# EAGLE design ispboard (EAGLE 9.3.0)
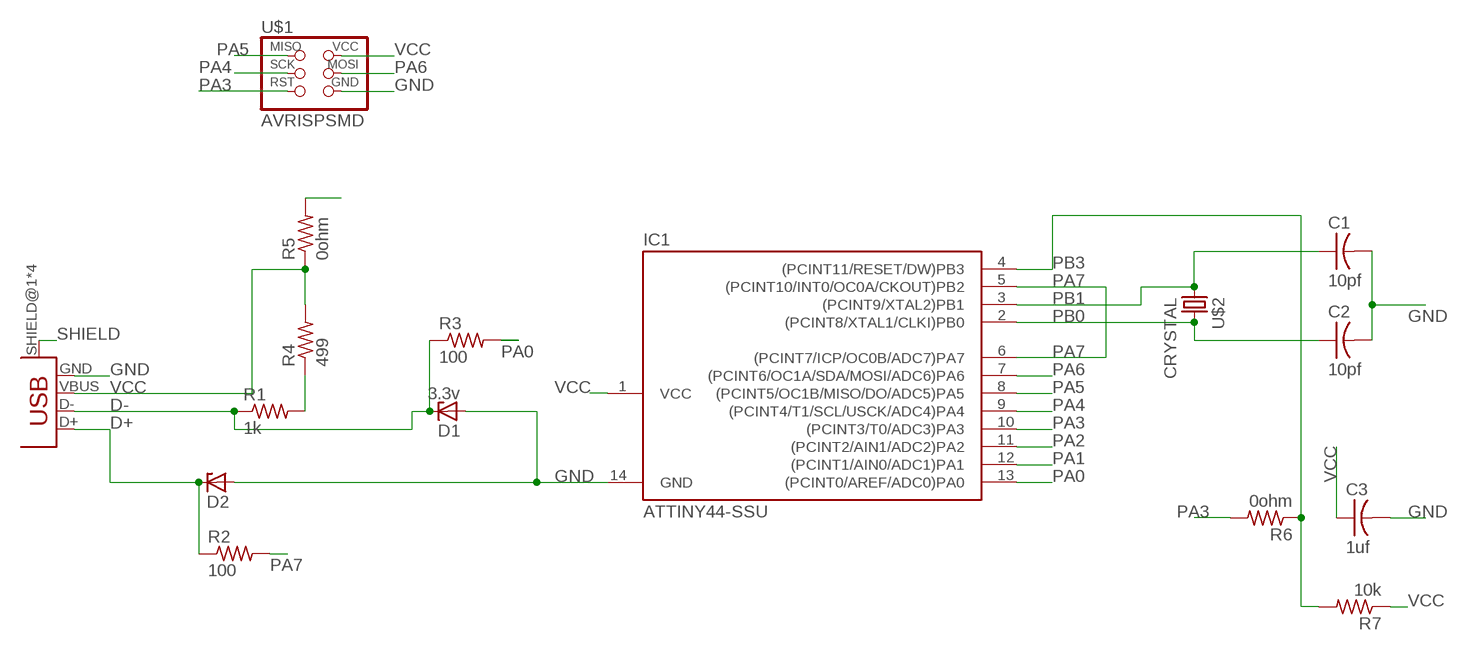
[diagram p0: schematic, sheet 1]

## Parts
C1  10pf  CAP-US1206FAB  [C1206FAB]
C2  10pf  CAP-US1206FAB  [C1206FAB]
C3  1uf  CAP-US1206FAB  [C1206FAB]
D1  3.3v  ZENER_DIODESOD123  [SOD123]
D2  ZENER_DIODESOD123  [SOD123]
IC1  ATTINY44-SSU  [SOIC14]
R1  1k  RES-US1206FAB  [R1206FAB]
R2  100  RES-US1206FAB  [R1206FAB]
R3  100  RES-US1206FAB  [R1206FAB]
R4  499  RES-US1206FAB  [R1206FAB]
R5  0ohm  RES-US1206FAB  [R1206FAB]
R6  0ohm  RES-US1206FAB  [R1206FAB]
R7  10k  RES-US1206FAB  [R1206FAB]
U$1  AVRISPSMD  [2X03SMD]
U$2  CRYSTAL  [2-SMD-5X3MM]
U$3  USB_MINIB  [USB_MINIB]

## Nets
D+: D2.CATHODE R2.1 U$3.D+
D-: D1.CATHODE R1.1 R3.1 U$3.D-
GND: C1.2 C2.2 C3.2 D1.ANODE D2.ANODE IC1.14(GND) U$1.6(GND) U$3.GND
N$1: R1.2 R4.1
PA0: IC1.13((PCINT0/AREF/ADC0)PA0) R3.2
PA1: IC1.12((PCINT1/AIN0/ADC1)PA1)
PA2: IC1.11((PCINT2/AIN1/ADC2)PA2)
PA3: IC1.10((PCINT3/T0/ADC3)PA3) R6.2 U$1.5(RST)
PA4: IC1.9((PCINT4/T1/SCL/USCK/ADC4)PA4) U$1.3(SCK)
PA5: IC1.8((PCINT5/OC1B/MISO/DO/ADC5)PA5) U$1.1(MISO)
PA6: IC1.7((PCINT6/OC1A/SDA/MOSI/ADC6)PA6) U$1.4(MOSI)
PA7: IC1.5((PCINT10/INT0/OC0A/CKOUT)PB2) IC1.6((PCINT7/ICP/OC0B/ADC7)PA7) R2.2
PB0: C2.1 IC1.2((PCINT8/XTAL1/CLKI)PB0) U$2.P$2
PB1: C1.1 IC1.3((PCINT9/XTAL2)PB1) U$2.P$1
PB3: IC1.4((PCINT11/RESET/DW)PB3) R6.1 R7.2
SHIELD: U$3.SHIELD@1(SHIELD) U$3.SHIELD@2(SHIELD) U$3.SHIELD@3(SHIELD) U$3.SHIELD@4(SHIELD)
VCC: C3.1 IC1.1(VCC) R4.2 R5.1 R5.2 R7.1 U$1.2(VCC) U$3.VBUS

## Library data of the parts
C1-C3 = fab:CAP-US
D1 D2 = fab:ZENER_DIODE: zener diode
IC1 = fab:ATTINY44
R1-R7 = fab:RES-US: Resistor (US Symbol)
U$1 = fab:AVRISP
U$2 = fab:CRYSTAL
U$3 = fab:USB_MINIB

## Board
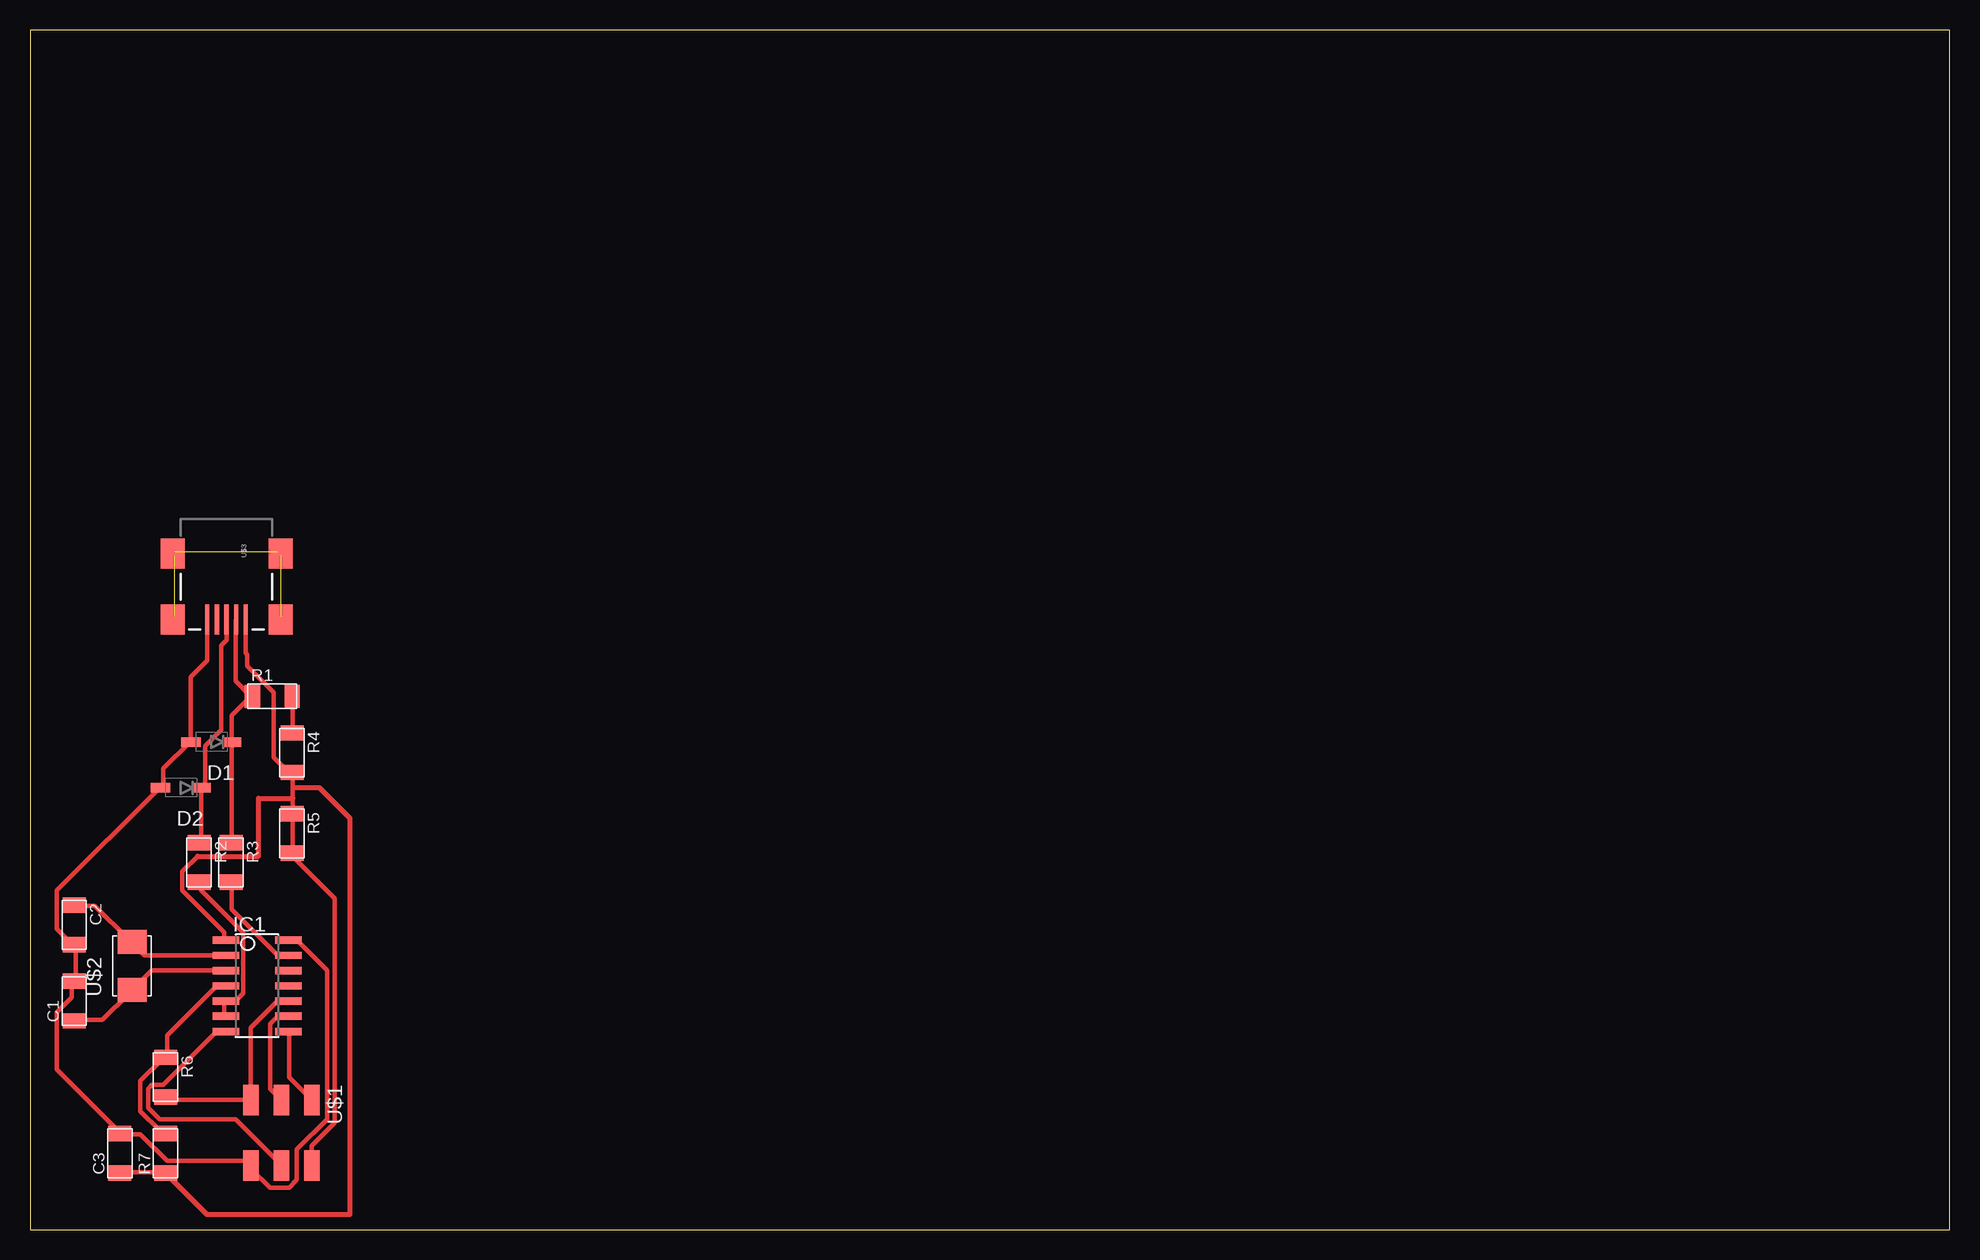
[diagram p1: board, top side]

Size 160 x 100 mm. Coordinates in mm from the lower left corner, seen from the top.
Outline: 0,0 160,0 160,100 0,100 0,0
Copper layers (1*16): Top 0.035mm / dielectric 1.5mm / Bottom 0.035mm
Design rules "default *": minimum track width 15mil, minimum drill 0.35mm, track to track 10mil, track to pad 6mil, pad to pad 6mil, via to via 6mil, smd to smd 6mil, copper to edge 40mil, drill to drill 6mil, minimum pad ring 10mil, minimum via ring 8mil, stop-mask expansion 4mil, vias tented up to drill 0mil, thermal gap 10mil

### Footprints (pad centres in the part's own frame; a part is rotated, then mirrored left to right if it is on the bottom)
C1206FAB = smd 1.27 x 1.905: 1 -1.651,0; 2 1.651,0
SOD123 = smd 1.6 x 0.8: ANODE 1.7,0; CATHODE -1.7,0
SOIC14 = smd 0.61 x 2.21: 1 -3.81,-2.603; 2 -2.54,-2.603; 3 -1.27,-2.603; 4 0,-2.603; 5 1.27,-2.603; 6 2.54,-2.603; 7 3.81,-2.603; 8 3.81,2.603; 9 2.54,2.603; 10 1.27,2.603; 11 0,2.603; 12 -1.27,2.603; 13 -2.54,2.603; 14 -3.81,2.603
R1206FAB = smd 1.27 x 1.905: 1 -1.651,0; 2 1.651,0
2X03SMD = smd 2.54 x 1.27: 1 -2.54,2.54; 2 2.92,2.54; 3 -2.54,0; 4 2.92,0; 5 -2.54,-2.54; 6 2.92,-2.54
2-SMD-5X3MM = smd 2 x 2.4: P$1 -2,0; P$2 2,0
USB_MINIB = smd 2.5 x 0.35: D+ 3.77,0; D- 3.77,0.8; GND 3.77,-1.6; ID 3.77,-0.8; VBUS 3.77,1.6 | smd 2.5 x 2: SHIELD@1 -1.73,-4.5; SHIELD@2 -1.73,4.5; SHIELD@3 3.77,4.5; SHIELD@4 3.77,-4.5

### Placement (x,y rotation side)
C1  3.68,19.05 90 top
C2  3.68,25.4 270 top
C3  7.49,6.35 90 top
D1  15.11,40.64 180 top
D2  12.57,36.83 180 top
IC1  18.92,20.32 270 top
R1  20.19,44.45 0 top
R2  14.1,30.61 270 top
R3  16.76,30.61 270 top
R4  21.84,39.75 270 top
R5  21.84,33.02 270 top
R6  11.3,12.7 270 top
R7  11.3,6.35 90 top
U$1  20.95,8.26 270 top
U$2  8.51,21.97 90 top
U$3  16.38,54.61 270 top

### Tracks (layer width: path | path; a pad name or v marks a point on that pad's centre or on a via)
D+
  Top 0.381: 14.29,36.83 14.29,32.38 R2.1 | 14.29,36.83 14.61,37.15 14.61,40.32 15.94,41.66 15.94,48.7 16.38,49.15 U$3.D+ | 14.29,36.83 D2.CATHODE
D-
  Top 0.381: 16.83,40.64 16.83,42.86 18.41,44.45 | 16.83,40.64 16.83,32.38 R3.1 | 16.83,40.64 D1.CATHODE | 18.41,44.45 17.14,45.72 17.14,50.8 U$3.D- | 18.41,44.45 R1.1
GND
  Top 0.381: D1.ANODE 13.34,40.64 11.11,38.42 11.11,36.83 D2.ANODE 10.79,36.83 2.22,28.26 2.22,25.08 3.49,23.81 C2.2 3.81,23.5 3.81,20.95 C1.2 3.49,20.64 3.49,19.37 2.22,18.1 2.22,13.34 7.3,8.26 C3.2 7.62,7.94 9.21,7.94 11.43,5.71 18.1,5.71 18.41,5.4 U$1.6 18.41,5.08 20,3.49 21.59,3.49 22.23,4.13 22.23,6.67 24.77,9.21 24.77,21.59 22.23,24.13 IC1.14 | 13.65,40.64 D1.ANODE | D1.ANODE 13.41,46.05 14.78,47.42 U$3.GND
N$1
  Top 0.381: R4.1 21.91,41.59 21.91,44.45 R1.2
PA0
  Top 0.381: IC1.13 20.64,22.86 16.83,26.67 16.83,28.89 R3.2
PA3
  Top 0.381: R6.2 11.43,10.79 U$1.5 18.41,16.83 20.64,19.05 IC1.10
PA4
  Top 0.381: IC1.9 20.64,17.78 20,17.14 20,11.75 U$1.3
PA5
  Top 0.381: U$1.1 21.59,12.7 21.59,16.51 IC1.8
PA6
  Top 0.381: IC1.7 15.56,16.51 11.11,12.06 10.16,12.06 9.84,11.75 9.84,10.16 10.79,9.21 17.14,9.21 20.95,5.4 U$1.4
PA7
  Top 0.381: R2.2 14.29,28.89 14.29,28.26 17.78,24.77 17.78,19.68 17.14,19.05 IC1.5 16.19,19.05 16.19,17.78 IC1.6
PB0
  Top 0.381: C2.1 3.81,26.99 5.4,26.99 8.26,24.13 U$2.P$2 8.57,23.81 9.53,22.86 IC1.2
PB1
  Top 0.381: C1.1 3.81,17.46 6.03,17.46 8.26,19.68 U$2.P$1 8.57,20 10.16,21.59 IC1.3
PB3
  Top 0.381: R7.2 11.11,8.26 10.79,8.26 9.21,9.84 9.21,12.38 11.11,14.29 R6.1 11.43,14.61 11.43,16.19 15.56,20.32 IC1.4
SHIELD  (3 unrouted)
  Top 0.381: 12.06,51.12 U$3.SHIELD@4 | 12.06,56.2 U$3.SHIELD@1 12.06,56.52 | 20.95,51.12 U$3.SHIELD@3 | 20.95,56.2 U$3.SHIELD@2 20.64,56.52
VCC
  Top 0.381: C3.1 7.62,4.76 11.11,4.76 R7.1 | 23.5,4.45 U$1.2 23.5,6.99 25.4,8.89 25.4,27.62 21.91,31.11 R5.2 | R5.2 21.91,31.43 21.91,34.61 R5.1 21.91,34.92 21.91,35.94 21.91,36.83 21.91,38.1 R4.2 21.59,38.1 20.32,39.37 20.32,44.77 18.1,46.99 18.1,47.94 17.98,48.06 U$3.VBUS | 13.97,31.11 12.7,29.84 12.7,28.26 16.19,24.77 16.19,24.13 IC1.1 | 21.59,31.11 R5.2
  Top 0.406: 13.97,31.11 19.05,31.11 19.05,35.94 21.91,35.94 | R7.1 14.73,1.27 26.67,1.27 26.67,34.29 24.13,36.83 21.91,36.83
